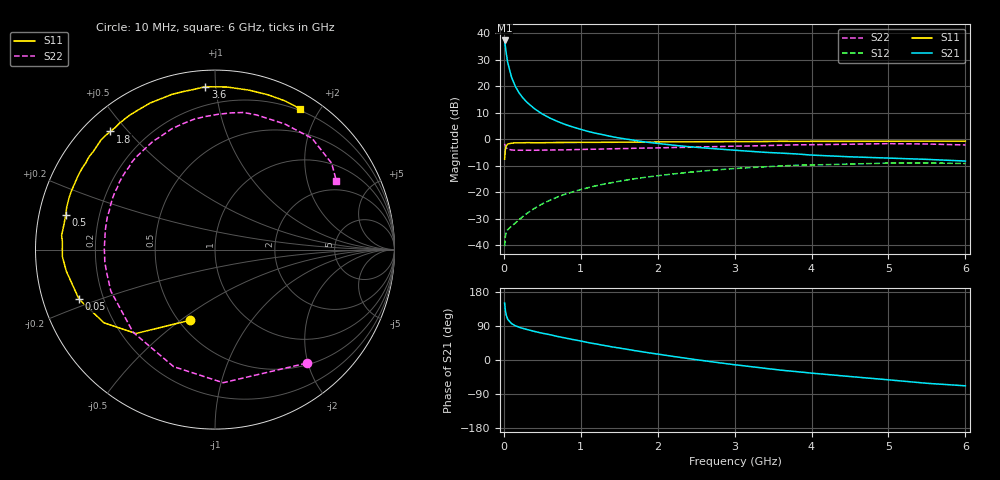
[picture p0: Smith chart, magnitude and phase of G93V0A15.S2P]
! SIEMENS Small Signal Semiconductors
! BFG235
! Si NPN RF Bipolar Junction Transistor in SOT223
! VCE = 3 V  IC = 150 mA
! Common Emitter S-Parameters:  July  1994
# GHz  S  MA  R  50
!  f  S11  S21  S12  S22
! GHz  MAG  ANG  MAG  ANG  MAG  ANG  MAG  ANG
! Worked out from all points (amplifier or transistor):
!   40 points, 10 MHz to 6 GHz, reference 50 ohm
!   highest |S21| = 37.2 dB at 10 MHz (marker M1)
!   |S21| within 3 dB of that: start of sweep to 22.95 MHz
!   unconditionally stable (mu >= 1): 423.6 MHz to 1.539 GHz
!   at 200 MHz: K = 0.82, MSG = 23.8 dB, |S12| = -30.3 dB
!   at 1.5 GHz: K = 1.01, MAG = 7.6 dB, |S12| = -15.9 dB
!   at 6 GHz: K = 0.91, MSG = 0.5 dB, |S12| = -9.2 dB
!   S11 on the Smith chart (normalised r, x): 10 MHz: 0.57, -0.54; 50 MHz: 0.11, -0.17; 500 MHz: 0.08, +0.11; 1.8 GHz: 0.08, +0.45; 3.6 GHz: 0.09, +0.94; 6 GHz: 0.18, +1.76
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0.01  0.418 -109.6  72.33 150.4  0.0096 60.8  0.8128 -51.1
0.02  0.6424 -133.3  55.3 130.9  0.0147 46.4  0.743 -86.5
0.03  0.7409 -146.6  42.62 119.3  0.0176 38.8  0.6916 -109.5
0.05  0.8065 -160.0  28 107.4  0.0196 33.3  0.6482 -134.8
0.1  0.8373 -171.8  14.67 96.1  0.0229 37.0  0.6247 -158.3
0.15  0.851 -177.3  9.833 90.3  0.0263 43.6  0.617 -168.0
0.2  0.8507 180.0  7.354 86.5  0.0305 48.5  0.6178 -173.5
0.25  0.8517 176.9  5.927 83.2  0.0351 51.8  0.6159 -177.4
0.3  0.8582 174.7  4.945 80.6  0.0398 55.0  0.6169 179.3
0.4  0.8529 170.3  3.725 75.3  0.0498 57.2  0.6165 174.4
0.5  0.8538 167.0  2.974 70.7  0.0602 58.2  0.6203 170.3
0.7  0.8631 160.2  2.146 62.0  0.0815 57.4  0.6271 162.9
0.9  0.8641 154.9  1.687 53.9  0.1017 54.4  0.6329 156.6
1.1  0.8684 148.5  1.389 45.8  0.1221 50.9  0.6427 150.4
1.4  0.8706 141.3  1.117 34.9  0.1509 44.7  0.6567 141.8
1.8  0.879 131.5  0.899 21.7  0.1873 35.9  0.6771 130.7
2.2  0.887 122.6  0.769 9.5  0.2204 26.8  0.6949 120.0
3.2  0.898 101.3  0.589 -17.2  0.2904 3.6  0.7434 94.1
3.6  0.9094 93.4  0.545 -26.8  0.3115 -6.2  0.7671 83.2
4.5  0.9084 77.8  0.464 -43.6  0.3385 -25.7  0.8006 61.0
5.5  0.9158 64.7  0.415 -61.5  0.3563 -47.2  0.8086 36.5
6  0.9168 58.8  0.386 -68.1  0.3463 -55.4  0.7762 29.3
